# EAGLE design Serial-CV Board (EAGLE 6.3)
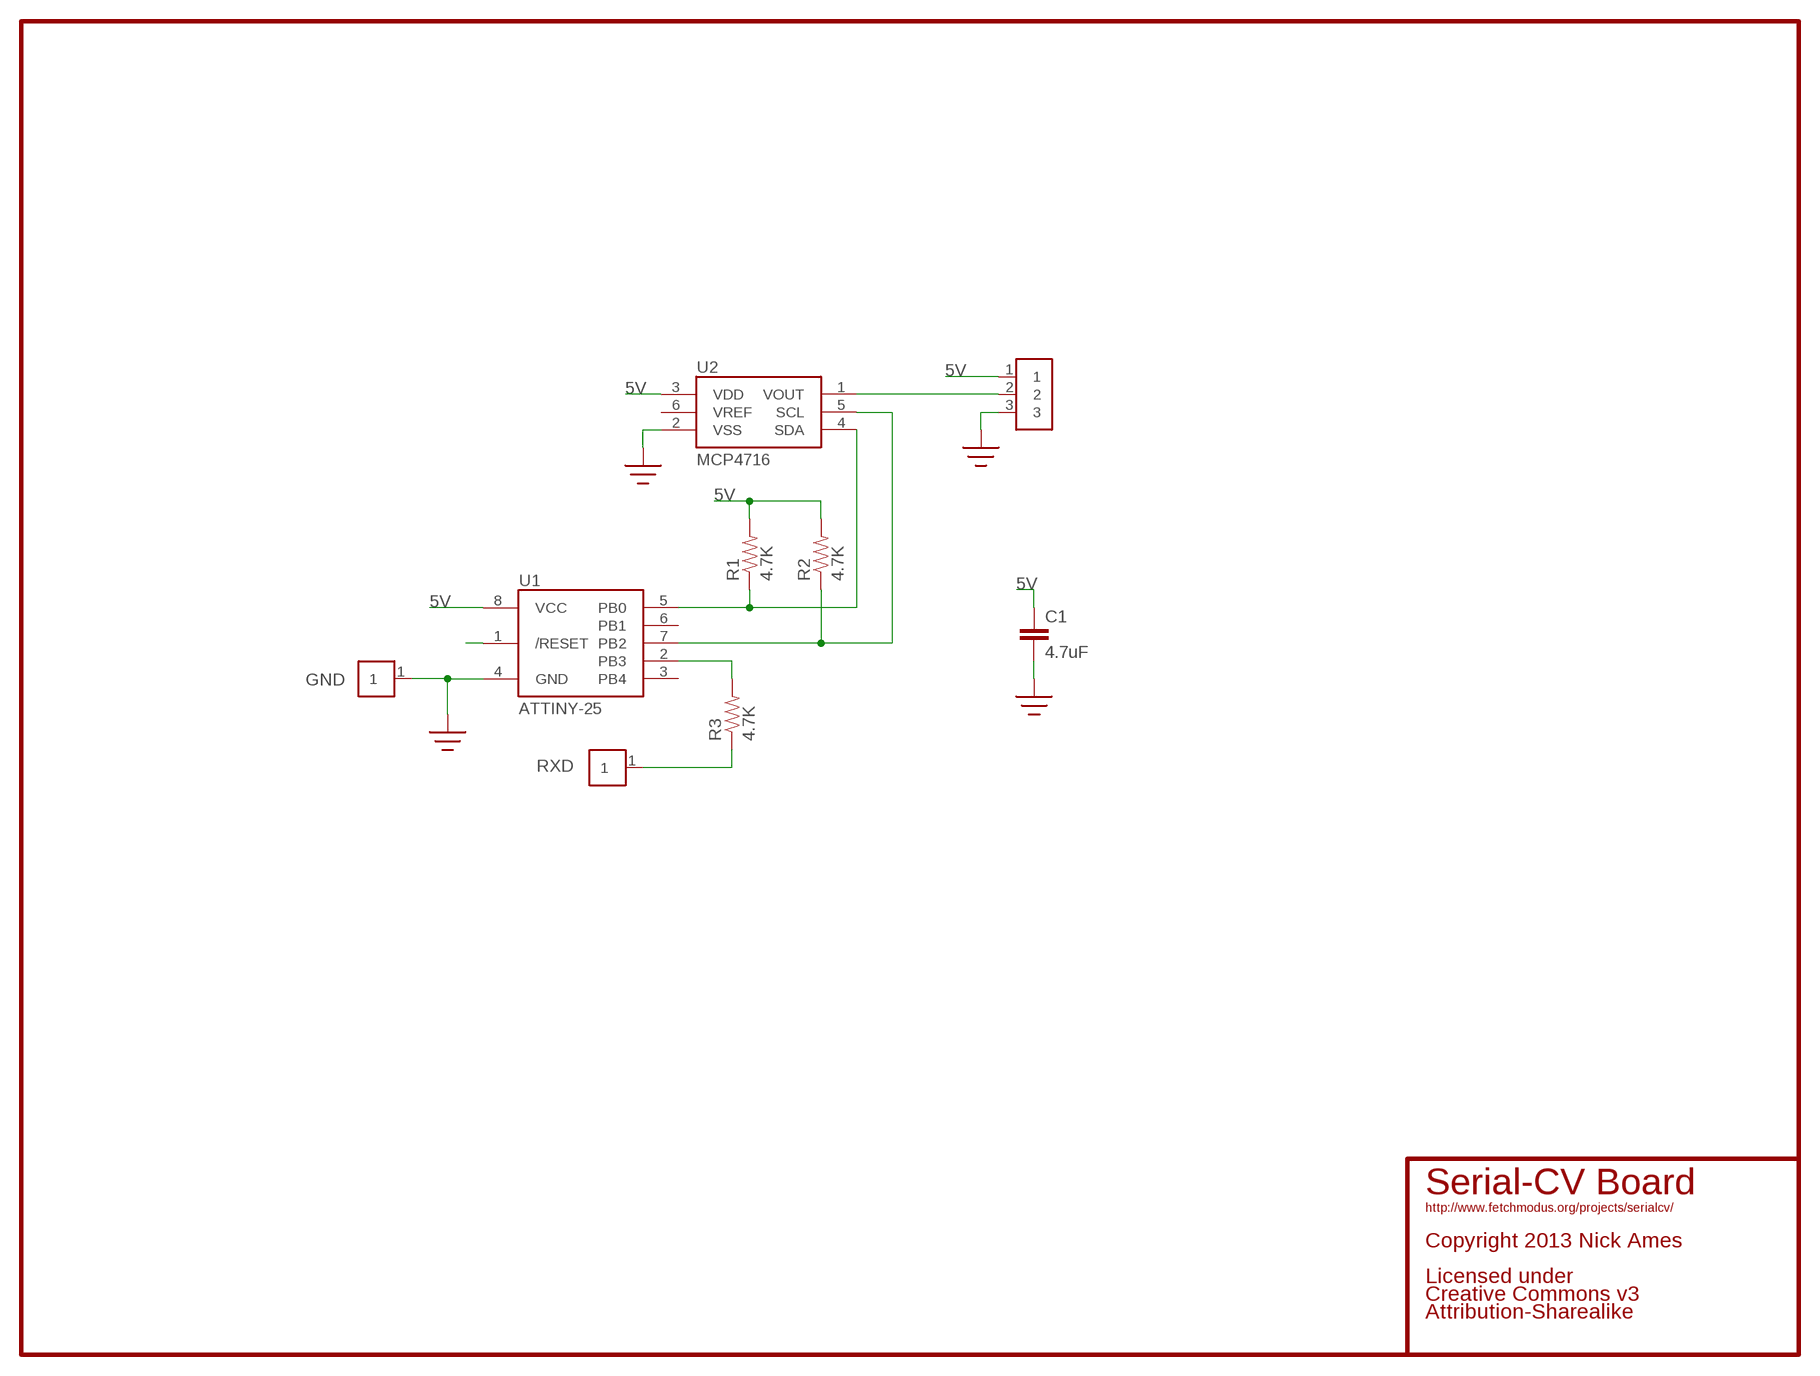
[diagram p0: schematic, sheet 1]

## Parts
C1  4.7uF  CAP0603-CAP  [0603-CAP]
JP1  HEADER-01  [HEADER-01]
JP2  HEADER-01  [HEADER-01]
R1  4.7K  RESISTOR0603-RES  [0603-RES]
R2  4.7K  RESISTOR0603-RES  [0603-RES]
R3  4.7K  RESISTOR0603-RES  [0603-RES]
U1  ATTINY-25  [SOIC8]
U2  MCP4716  [SOT-23-6]
U$5  HEADER-03  [HEADER-03]

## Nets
5V: C1.1 R1.2 R2.2 U1.8(VCC) U2.3(VDD) U$5.1
GND: C1.2 JP1.1 U1.4(GND) U2.2(VSS) U$5.3
N$1: JP2.1 R3.1
N$2: U2.1(VOUT) U$5.2
N$4: R3.2 U1.2(PB3)
N$5: U1.1(/RESET)
SCL: R1.1 U1.5(PB0) U2.4(SDA)
SDA: R2.1 U1.7(PB2) U2.5(SCL)
Unconnected: U1.3(PB4) U1.6(PB1) U2.6(VREF)

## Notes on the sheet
- GND
- RXD
- Serial-CV Board
- http://www.fetchmodus.org/projects/serialcv/
- Copyright 2013 Nick Ames
- Licensed under
- Creative Commons v3
- Attribution-Sharealike

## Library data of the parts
C1 = SparkFun:CAP: Capacitor
JP1 JP2 = NA-lib:HEADER-01
R1-R3 = SparkFun:RESISTOR: Resistor
U1 = NA-lib:ATTINY-25
U2 = NA-lib:MCP4716
U$5 = NA-lib:HEADER-03

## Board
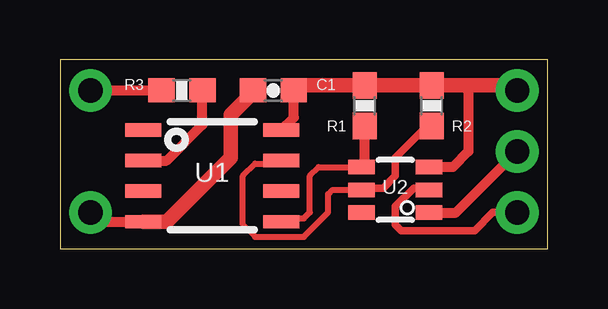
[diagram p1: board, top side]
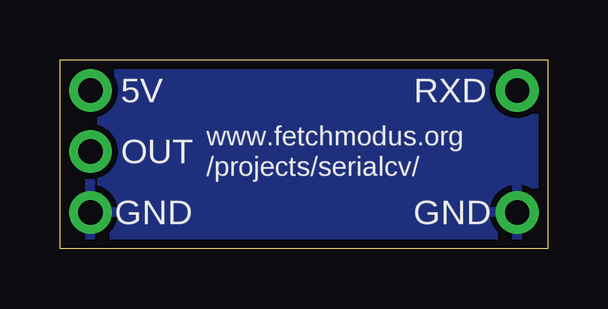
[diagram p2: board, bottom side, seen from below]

Size 20.32 x 7.87 mm. Coordinates in mm from the lower left corner, seen from the top.
Outline: 0,0 20.32,0 20.32,7.87 0,7.87 0,0
Copper layers (1*16): Top 0.0356mm / dielectric 1.5011mm / Bottom 0.0356mm
Design rules "LaenPCBOrder *": minimum track width 6mil, minimum drill 13mil, track to track 6mil, track to pad 6mil, pad to pad 6mil, via to via 6mil, smd to smd 6mil, copper to edge 15mil, drill to drill 6mil, minimum pad ring 7mil, minimum via ring 7mil, stop-mask expansion 4mil, vias tented up to drill 30mil, thermal gap 10mil

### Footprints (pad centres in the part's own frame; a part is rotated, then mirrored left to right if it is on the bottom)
0603-CAP = smd 1.1 x 1: 1 -0.85,0; 2 0.85,0
HEADER-01 = drill 1.016 pad 1.778: 1 0,0
0603-RES = smd 1.1 x 1: 1 -0.85,0; 2 0.85,0
SOIC8 = smd 1.5 x 0.55: 1 -2.875,1.91; 2 -2.875,0.635; 3 -2.875,-0.635; 4 -2.875,-1.91; 5 2.875,-1.91; 6 2.875,-0.635; 7 2.875,0.635; 8 2.875,1.91
SOT-23-6 = smd 1.1 x 0.6: 1 -1.4,0.95; 2 -1.4,0; 3 -1.4,-0.95; 4 1.4,-0.95; 5 1.4,0; 6 1.4,0.95
HEADER-03 = drill 1.016 pad 1.778: 1 0,2.54; 2 0,0; 3 0,-2.54

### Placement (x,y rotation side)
C1  8.89,6.6 180 top
JP1  1.27,1.52 0 top
JP2  1.27,6.6 0 top
R1  12.7,5.97 90 top
R2  15.49,5.97 90 top
R3  5.08,6.6 0 top
U1  6.35,3.05 0 top
U2  13.97,2.46 180 top
U$5  19.05,4.06 0 top

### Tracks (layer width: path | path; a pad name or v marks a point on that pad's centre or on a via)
5V
  Top 0.406: U2.3 16.37,3.41 17.02,4.06 17.02,6.57 16.76,6.82 | U1.8 9.74,5.47 C1.1
  Top 0.61: C1.1 9.96,6.82 R1.2 R2.2 16.76,6.82 18.84,6.82 U$5.1
GND
  Top 0.305: U$5.3 18.03,1.52 17.27,0.76 14.22,0.76 13.97,1.02 13.97,1.78 14.73,2.54 15.29,2.54 U2.2
  Top 0.406: JP1.1 1.66,1.14 U1.4
  Top 0.61: U1.4 4.44,1.14 7.11,3.81 7.11,5.59 8.04,6.52 C1.2
  pour Bottom (isolate 0.254): 0,7.87 20.32,7.87 20.32,0 0,0 0,7.62
N$1
  Top 0.406: JP2.1 R3.1
N$2
  Top 0.406: U2.1 16.5,1.51 U$5.2
N$4
  Top 0.406: R3.2 5.93,5.17 4.45,3.68 U1.2
SCL
  Top 0.254: U2.4 10.78,3.41 10.41,3.05 10.41,1.52 10.16,1.27 9.36,1.27 U1.5
  Top 0.406: R1.1 12.7,3.54 U2.4
SDA
  Top 0.254: U2.5 11.35,2.46 11.18,2.29 11.18,1.52 10.16,0.51 8.13,0.51 7.62,1.02 7.62,3.05 8.13,3.56 9.1,3.56 U1.7
  Top 0.305: R2.1 15.28,5.12 13.97,3.81 13.97,3.05 13.46,2.54 12.65,2.54 U2.5

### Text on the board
bPlace: RXD | 5V | www.fetchmodus.org | OUT | /projects/serialcv/ | GND | GND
